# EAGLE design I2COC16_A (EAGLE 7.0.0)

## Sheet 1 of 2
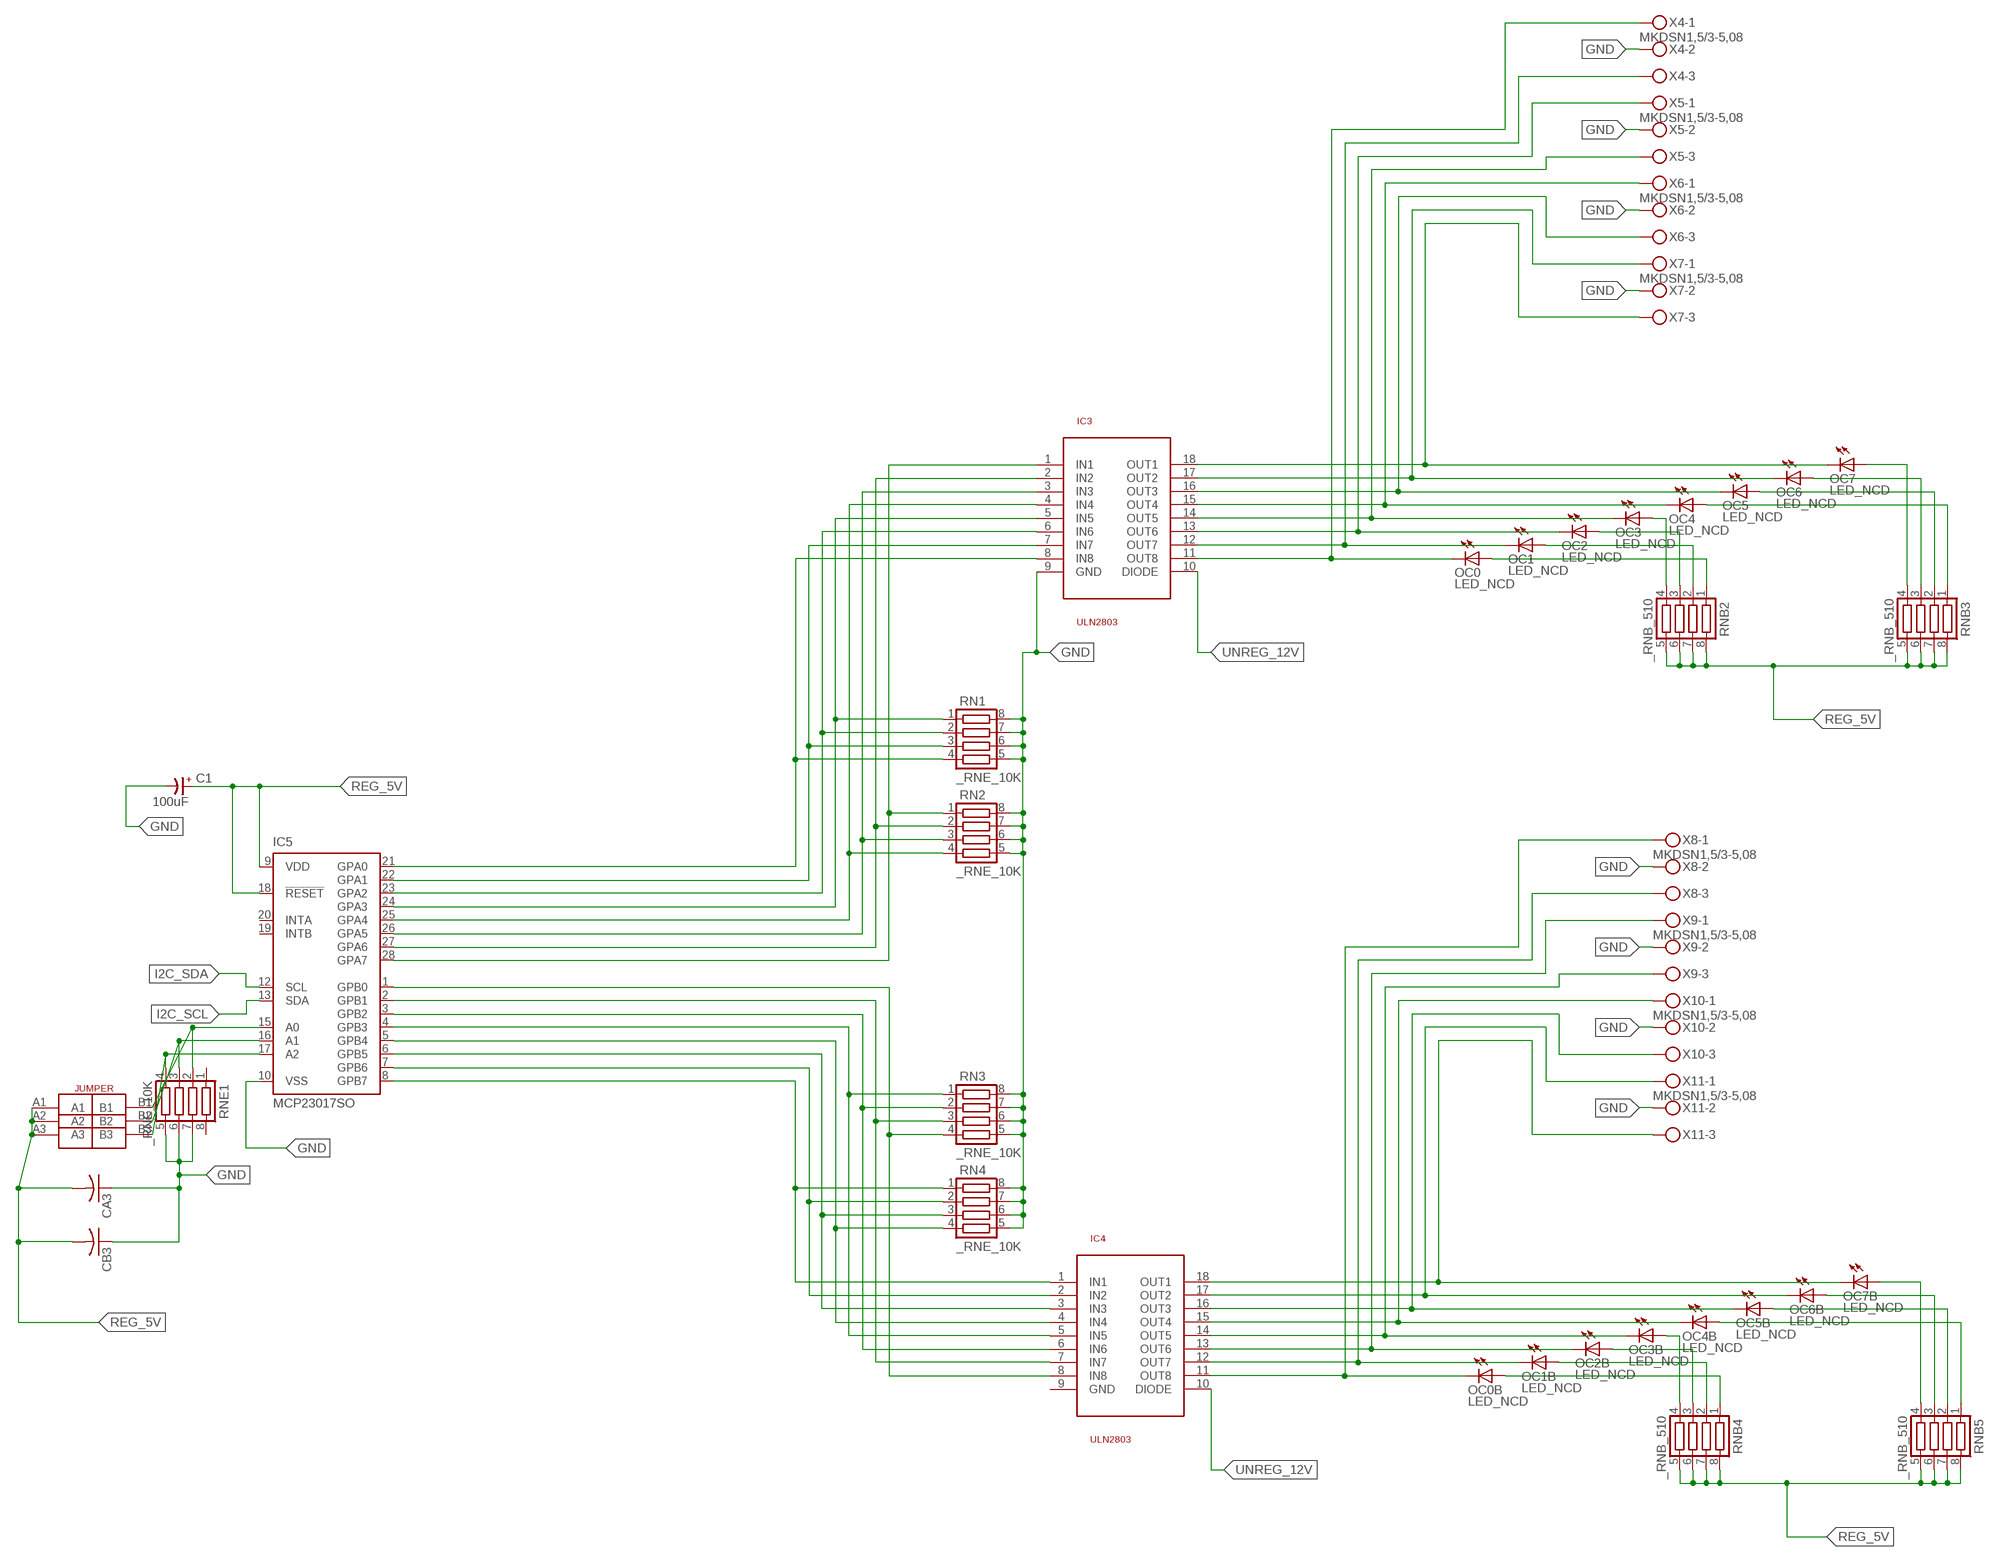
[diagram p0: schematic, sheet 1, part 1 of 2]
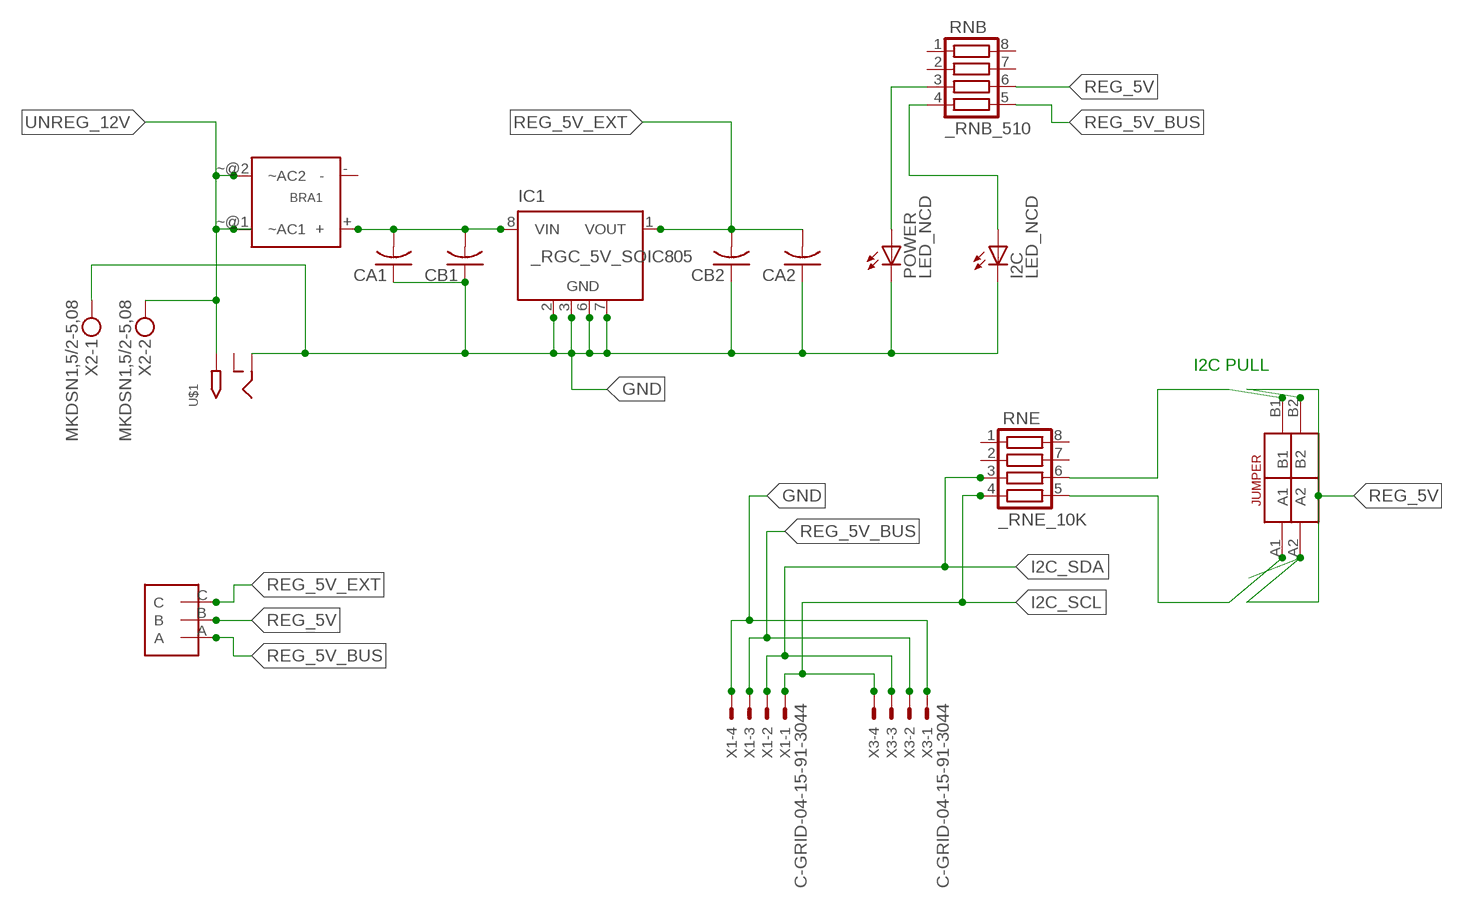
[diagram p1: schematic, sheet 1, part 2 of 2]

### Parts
BRA1  MB2S_  [MB2S]
C1  100uF  CP-E-025X060  [E-025X060]
CA1  CC1206KRX7R9BB104C1206K  [CC1206KRX7R9BB104]
CA2  CC1206KRX7R9BB104C1206K  [CC1206KRX7R9BB104]
CA3  CC1206KRX7R9BB104C1206K  [CC1206KRX7R9BB104]
CB1  TMK316F106ZL-TC1206K  [TMK316F106ZL-T]
CB2  TMK316F106ZL-TC1206K  [TMK316F106ZL-T]
CB3  TMK316F106ZL-TC1206K  [TMK316F106ZL-T]
I2C  LED_NCD  [CHIPLED_0603]
IC1  _RGC_5V_SOIC805  [_RGC_5V_SOIC8]
IC3  ULN2803  [SO18L]
IC4  ULN2803  [SO18L]
IC5  MCP23017SO  [SO28W]
OC0  LED_NCD  [CHIPLED_0603]
OC0B  LED_NCD  [CHIPLED_0603]
OC1  LED_NCD  [CHIPLED_0603]
OC1B  LED_NCD  [CHIPLED_0603]
OC2  LED_NCD  [CHIPLED_0603]
OC2B  LED_NCD  [CHIPLED_0603]
OC3  LED_NCD  [CHIPLED_0603]
OC3B  LED_NCD  [CHIPLED_0603]
OC4  LED_NCD  [CHIPLED_0603]
OC4B  LED_NCD  [CHIPLED_0603]
OC5  LED_NCD  [CHIPLED_0603]
OC5B  LED_NCD  [CHIPLED_0603]
OC6  LED_NCD  [CHIPLED_0603]
OC6B  LED_NCD  [CHIPLED_0603]
OC7  LED_NCD  [CHIPLED_0603]
OC7B  LED_NCD  [CHIPLED_0603]
POWER  LED_NCD  [CHIPLED_0603]
RN1  _RNE_10K  [RNE]
RN2  _RNE_10K  [RNE]
RN3  _RNE_10K  [RNE]
RN4  _RNE_10K  [RNE]
RNB  _RNB_510  [RNB]
RNB2  _RNB_510  [RNB]
RNB3  _RNB_510  [RNB]
RNB4  _RNB_510  [RNB]
RNB5  _RNB_510  [RNB]
RNE  _RNE_10K  [RNE]
RNE1  _RNE_10K  [RNE]
U$1  2.1MMJACK  [PJ-102A]
U$2  JUMPER_1X3  [JUMPER_1X3]
U$3  JUMPER_2X2  [JUMPER_2X2]
U$18  JUMPER_3X2  [JUMPER_3X2]
X1  C-GRID-04-15-91-3044  [15-91-04]
X2  MKDSN1,5/2-5,08  [MKDSN1,5/2-5,08]
X3  C-GRID-04-15-91-3044  [15-91-04]
X4  MKDSN1,5/3-5,08  [MKDSN1,5/3-5,08]
X5  MKDSN1,5/3-5,08  [MKDSN1,5/3-5,08]
X6  MKDSN1,5/3-5,08  [MKDSN1,5/3-5,08]
X7  MKDSN1,5/3-5,08  [MKDSN1,5/3-5,08]
X8  MKDSN1,5/3-5,08  [MKDSN1,5/3-5,08]
X9  MKDSN1,5/3-5,08  [MKDSN1,5/3-5,08]
X10  MKDSN1,5/3-5,08  [MKDSN1,5/3-5,08]
X11  MKDSN1,5/3-5,08  [MKDSN1,5/3-5,08]

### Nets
GND: C1.- CA1.1 CA2.1 CA3.1 CB1.1 CB2.1 CB3.1 I2C.C IC1.2(GND) IC1.3(GND) IC1.6(GND) IC1.7(GND) IC3.9(GND) IC5.10(VSS) POWER.C RN1.5 RN1.6 RN1.7 RN1.8 RN2.5 RN2.6 RN2.7 RN2.8 RN3.5 RN3.6 RN3.7 RN3.8 RN4.5 RN4.6 RN4.7 RN4.8 RNE1.5 RNE1.6 RNE1.7 U$1.RING X1.4 X2.1 X3.1 X4.2 X5.2 X6.2 X7.2 X8.2 X9.2 X10.2 X11.2
I2C_SCL: IC5.13(SDA) RNE.4 X1.1 X3.4
I2C_SDA: IC5.12(SCL) RNE.3 X1.2 X3.3
N$1: BRA1.+ CA1.2 CB1.2 IC1.8(VIN)
N$2: POWER.A RNB.3
N$3: I2C.A RNB.4
N$4: RNE.5 U$3.A1
N$5: RNE.6 U$3.B1
N$6: IC5.15(A0) RNE1.2 U$18.B1
N$7: IC5.16(A1) RNE1.3 U$18.B2
N$8: IC5.17(A2) RNE1.4 U$18.B3
N$9: IC3.11(OUT8) OC0.C X4.1
N$10: IC3.12(OUT7) OC1.C X4.3
N$11: IC3.13(OUT6) OC2.C X5.1
N$12: IC3.14(OUT5) OC3.C X5.3
N$13: IC3.1(IN1) IC5.28(GPA7) RN2.1
N$14: IC3.16(OUT3) OC5.C X6.3
N$15: IC3.17(OUT2) OC6.C X7.1
N$16: IC3.18(OUT1) OC7.C X7.3
N$17: IC3.2(IN2) IC5.27(GPA6) RN2.2
N$18: IC3.3(IN3) IC5.26(GPA5) RN2.3
N$19: IC3.4(IN4) IC5.25(GPA4) RN2.4
N$20: IC3.5(IN5) IC5.24(GPA3) RN1.1
N$21: IC3.6(IN6) IC5.23(GPA2) RN1.2
N$22: IC3.7(IN7) IC5.22(GPA1) RN1.3
N$23: IC3.8(IN8) IC5.21(GPA0) RN1.4
N$24: IC3.15(OUT4) OC4.C X6.1
N$25: OC7.A RNB3.4
N$26: OC6.A RNB3.3
N$27: OC5.A RNB3.2
N$28: OC4.A RNB3.1
N$29: OC3.A RNB2.4
N$30: OC2.A RNB2.3
N$31: OC1.A RNB2.2
N$32: OC0.A RNB2.1
N$33: IC4.11(OUT8) OC0B.C X8.1
N$34: IC4.12(OUT7) OC1B.C X8.3
N$35: IC4.13(OUT6) OC2B.C X9.1
N$36: IC4.14(OUT5) OC3B.C X9.3
N$37: IC4.16(OUT3) OC5B.C X10.3
N$38: IC4.17(OUT2) OC6B.C X11.1
N$39: IC4.18(OUT1) OC7B.C X11.3
N$40: IC4.15(OUT4) OC4B.C X10.1
N$41: OC7B.A RNB5.4
N$42: OC6B.A RNB5.3
N$43: OC5B.A RNB5.2
N$44: OC4B.A RNB5.1
N$45: OC3B.A RNB4.4
N$46: OC2B.A RNB4.3
N$47: OC1B.A RNB4.2
N$48: OC0B.A RNB4.1
N$49: IC4.1(IN1) IC5.8(GPB7) RN4.1
N$50: IC4.2(IN2) IC5.7(GPB6) RN4.2
N$51: IC4.3(IN3) IC5.6(GPB5) RN4.3
N$52: IC4.4(IN4) IC5.5(GPB4) RN4.4
N$53: IC4.5(IN5) IC5.4(GPB3) RN3.1
N$54: IC4.6(IN6) IC5.3(GPB2) RN3.2
N$55: IC4.7(IN7) IC5.2(GPB1) RN3.3
N$56: IC4.8(IN8) IC5.1(GPB0) RN3.4
REG_5V: C1.+ CA3.2 CB3.2 IC5.9(VDD) IC5.18(!RESET) RNB2.5 RNB2.6 RNB2.7 RNB2.8 RNB3.5 RNB3.6 RNB3.7 RNB3.8 RNB4.5 RNB4.6 RNB4.7 RNB4.8 RNB5.5 RNB5.6 RNB5.7 RNB5.8 RNB.6 U$2.B U$3.A2 U$3.B2 U$18.A1 U$18.A2 U$18.A3
REG_5V_BUS: RNB.5 U$2.A X1.3 X3.2
REG_5V_EXT: CA2.2 CB2.2 IC1.1(VOUT) U$2.C
UNREG_12V: BRA1.~@1(~AC1) BRA1.~@2(~AC2) IC3.10(DIODE) IC4.10(DIODE) U$1.TIP X2.2
Unconnected: BRA1.- IC1.4(NC) IC1.5(NC) IC4.9(GND) IC5.19(INTB) IC5.20(INTA) RNB.1 RNB.2 RNB.7 RNB.8 RNE1.1 RNE1.8 RNE.1 RNE.2 RNE.7 RNE.8 U$1.RING_SW

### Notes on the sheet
- I2C PULL

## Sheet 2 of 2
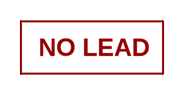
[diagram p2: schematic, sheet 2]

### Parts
U$16  NOPB_LOGO_SYM  [NOPB_LOGO_SYM]

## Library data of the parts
BRA1 = NCD_ULTIMATE_LIBRARY:MB2S: Bridge Rectifier BRA MB2S 200V 500ma Digikey MB2S-TPMSTR-ND/MB2S-TP
C1 = NCD_ULTIMATE_LIBRARY:CP-: Capacitors All Kinds POLARIZED CAP
CA1-CA3 = NCD_ULTIMATE_LIBRARY:CC1206KRX7R9BB104: Capacitor CA .1uF 50V SMT C1206K CC1206KRX7R9BB104
CB1-CB3 = NCD_ULTIMATE_LIBRARY:TMK316F106ZL-T: Capacitor CB 10uF SMT 1206 TMK316F106ZL-T
I2C POWER = NCD_ULTIMATE_bhaskar:LED_NCD
IC1 = NCD_ULTIMATE_LIBRARY:_RGC_5V_SOIC8: Regulator Linear 5V Chip Positive VOLTAGE REGULATOR Digikey 497-7267-2-ND/L78L05CD13TR
IC3 IC4 = NCD_ULTIMATE_LIBRARY:ULN2803: Semiconductor 8 O.C. N-Channel Transistor Driver Digikey ULN2803AFWGCELTR-ND/ULN2803AFWG,C,EL
IC5 = NCD_ULTIMATE_LIBRARY:MCP23017: Semiconductor Port Expander I/O 16-Bit I2C http://ww1.microchip.com/downloads/en/DeviceDoc/21952a.pdf Source: http://ww1.microchip.com/downloads/en/DeviceDoc/21952a.pdf
OC0 OC0B OC1 OC1B OC2 OC2B OC3 OC3B OC4 OC4B OC5 OC5B OC6 OC6B OC7 OC7B = NCD_ULTIMATE_LIBRARY:LED_NCD: LED Digikey 754-1132-2-ND/APT2012SRCPRV
RN1-RN4 RNE RNE1 = NCD_ULTIMATE_LIBRARY:_RNE_10K: Resistor Array RNE SMT 10K x 4 Single Resistor Source: http://www.ctscorp.com/components/Datasheets/CTSChipArrayDs.pdf Digikey 742C083103JPTR-ND/742C083103JP; OC_FARNELL: unknown; OC_NEWARK: unknown
RNB RNB2-RNB5 = NCD_ULTIMATE_LIBRARY:_RNB_510: Resistor Array RNB SMT 510 x 4 Single Resistor Source: http://www.ctscorp.com/components/Datasheets/CTSChipArrayDs.pdf Digikey 742C083511JPTR-ND/ 742C083511JP; OC_FARNELL: unknown; OC_NEWARK: unknown
U$1 = NCD_ULTIMATE_CONNECTORS:2.1MMJACK: 2.1mm x 5.5mm DC jack with internal switch. Digikey part #PJ-102A, 4UCON part #05537 By microbuilder.eu
U$2 = NCD_ULTIMATE_CONNECTORS:JUMPER_1X3
U$3 = NCD_ULTIMATE_CONNECTORS:JUMPER_2X2
U$16 = PatternAgents-Logos:NOPB_LOGO_SYM: NOPB_LOGO_SYM
U$18 = NCD_ULTIMATE_CONNECTORS:JUMPER_3X2
X1 X3 = NCD_ULTIMATE_CONNECTORS:C-GRID-04: CONNECTOR 4-Pos I2C wire to board 2.54 mm (0.100") pitch header Digikey WM1342-ND/0015912045; OC_FARNELL: unknown; OC_NEWARK: unknown
X2 = NCD_ULTIMATE_CONNECTORS:MKDSN1,5/2-5,08: MKDSN 1,5/ 2-5,08 Printklemme
X4-X11 = NCD_ULTIMATE_CONNECTORS:MKDSN1,5/3-5,08: MKDSN 1,5/ 3-5,08 Printklemme Nennstrom: 13,5 A Nennspannung: 250 V Rastermaß: 5,08 mm Polzahl: 3 Anschlussart: Schraubanschluss Montage: Löten Anschlussrichtung Leiter/Platine: 0 ° Artikelnummer: 1729131 Source: http://eshop.phoenixcontact.com .. 1729131.pdf

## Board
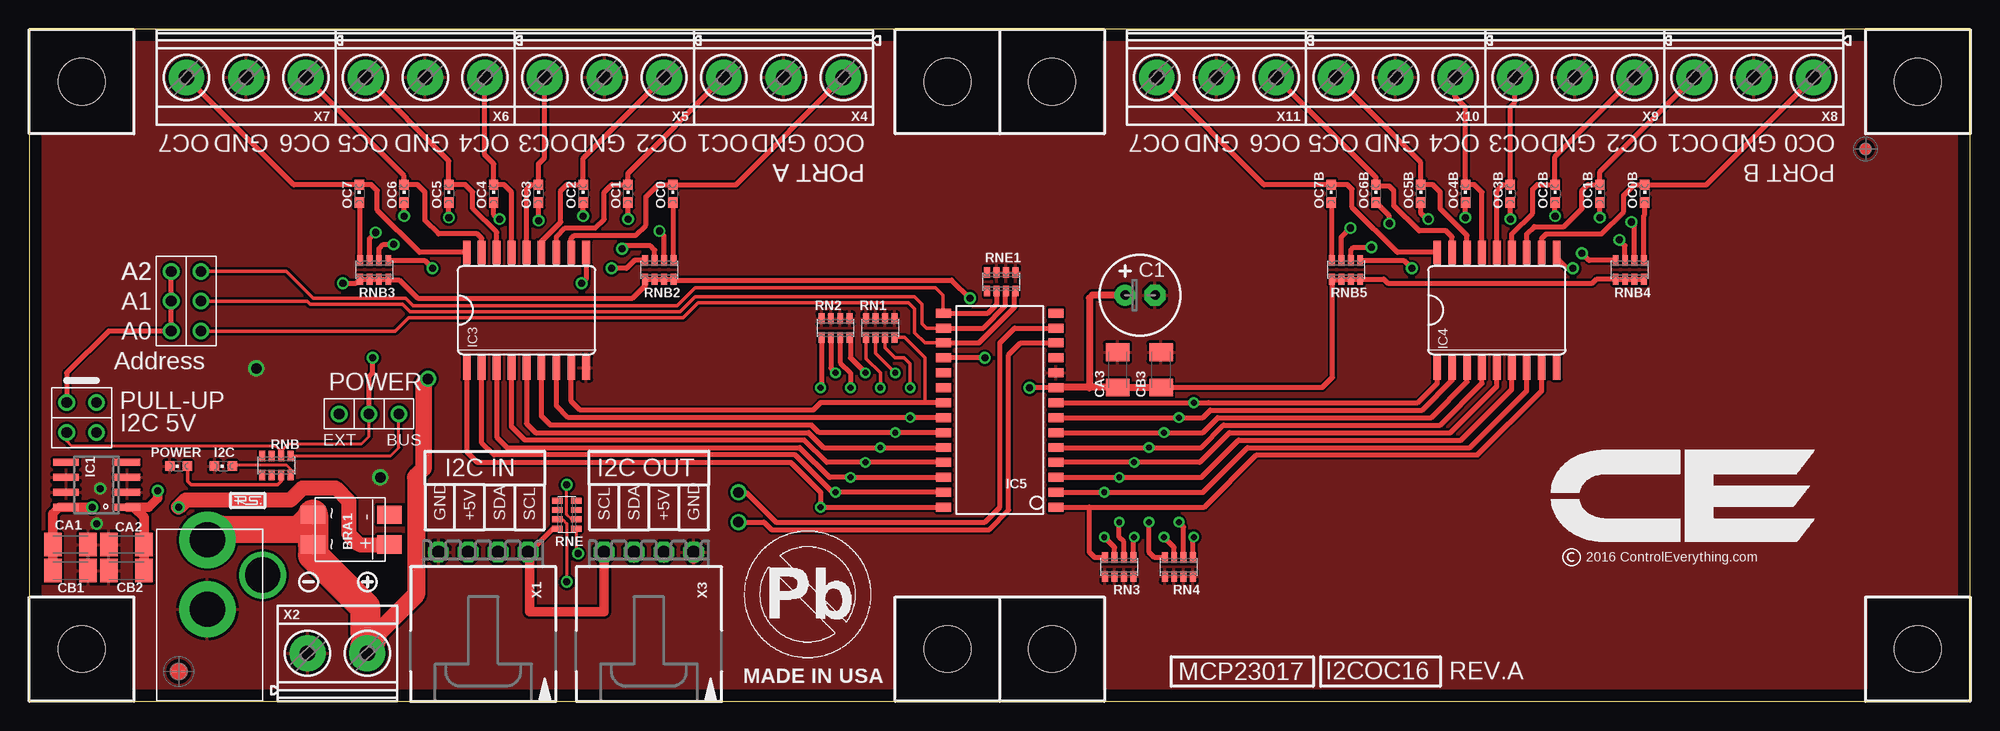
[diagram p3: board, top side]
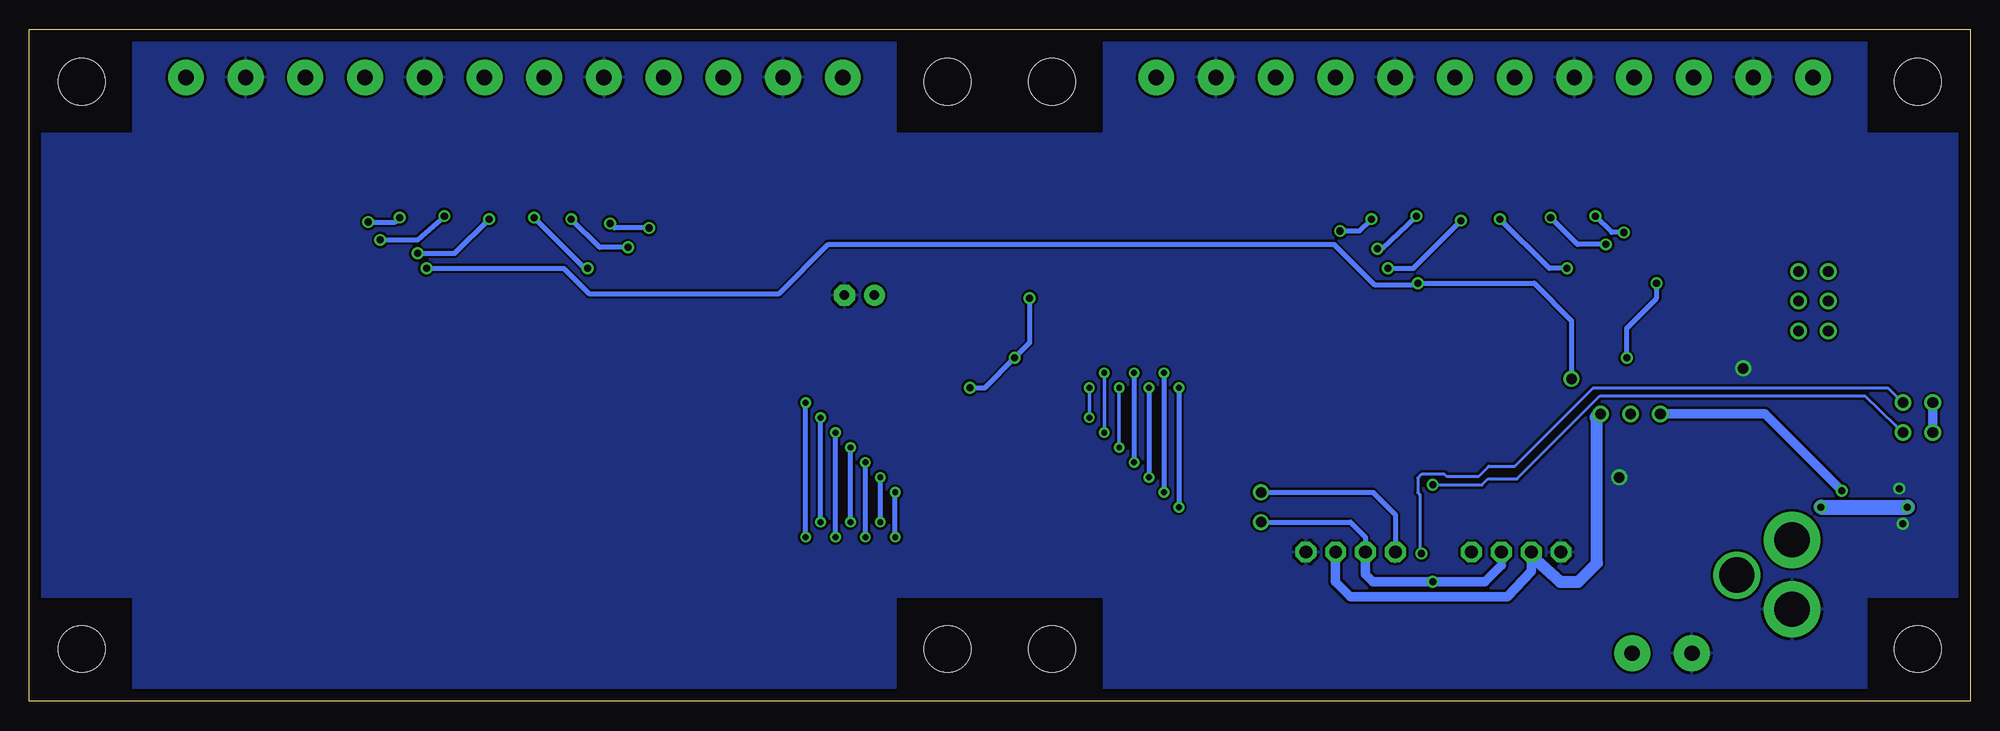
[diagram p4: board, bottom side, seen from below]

Size 165.1 x 57.15 mm. Coordinates in mm from the lower left corner, seen from the top.
Outline: 81.28,0 0,0 0,55.88
Outline: 81.28,0 82.53,0
Outline: 0,56.82 0,55.88
Outline: 81.28,0 82.55,0 163.83,0
Outline: 0,55.88 0,57.15 165.1,57.15 165.1,0 163.83,0
Outline: 163.83,0 165.08,0
Copper layers (1*16): Top 0.035mm / dielectric 1.5mm / Bottom 0.035mm
Design rules "default": minimum track width 10mil, minimum drill 24mil, track to track 8mil, track to pad 8mil, pad to pad 8mil, via to via 8mil, smd to smd 8mil, copper to edge 40mil, drill to drill 8mil, minimum pad ring 10mil, minimum via ring 8mil, stop-mask expansion 4mil, vias tented up to drill 0mil, thermal gap 10mil
Holes 3.96 mm at 4.45,4.45 78.11,4.45 78.11,52.7 4.45,52.7 87,52.7 87,4.45 160.66,4.45 160.66,52.7

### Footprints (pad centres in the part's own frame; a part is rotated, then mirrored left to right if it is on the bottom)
MB2S = smd 1.55 x 2.1: + 0,-6.5; - 2.54,-6.5; ~@1 0,0; ~@2 2.54,0
E-025X060 = drill 0.813 pad 1.778: + -1.27,0 | drill 0.813 pad 1.778 octagon: - 1.27,0
CC1206KRX7R9BB104 = smd 1.5 x 2: 1 -1.5,0; 2 1.5,0
TMK316F106ZL-T = smd 1.5 x 2: 1 -1.5,0; 2 1.5,0
CHIPLED_0603 = smd 0.8 x 0.8: A 0,-0.75; C 0,0.75
_RGC_5V_SOIC8 = smd 0.6 x 2.2: 1 -1.905,-2.6; 2 -0.635,-2.6; 3 0.635,-2.6; 4 1.905,-2.6; 5 1.905,2.6; 6 0.635,2.6; 7 -0.635,2.6; 8 -1.905,2.6
SO18L = smd 0.66 x 2.032: 1 -5.08,-4.902; 2 -3.81,-4.902; 3 -2.54,-4.902; 4 -1.27,-4.902; 5 0,-4.902; 6 1.27,-4.902; 7 2.54,-4.902; 8 3.81,-4.902; 9 5.08,-4.902; 10 5.08,4.902; 11 3.81,4.902; 12 2.54,4.902; 13 1.27,4.902; 14 0,4.902; 15 -1.27,4.902; 16 -2.54,4.902; 17 -3.81,4.902; 18 -5.08,4.902
SO28W = smd 0.762 x 1.27: 1 -7.62,-4.78; 2 -6.35,-4.78; 3 -5.08,-4.78; 4 -3.81,-4.78; 5 -2.54,-4.78; 6 -1.27,-4.78; 7 0,-4.78; 8 1.27,-4.78; 9 2.54,-4.78; 10 3.81,-4.78; 11 5.08,-4.78; 12 6.35,-4.78; 13 7.62,-4.78; 14 8.89,-4.78; 15 8.89,4.78; 16 7.62,4.78; 17 6.35,4.78; 18 5.08,4.78; 19 3.81,4.78; 20 2.54,4.78; 21 1.27,4.78; 22 0,4.78; 23 -1.27,4.78; 24 -2.54,4.78; 25 -3.81,4.78; 26 -5.08,4.78; 27 -6.35,4.78; 28 -7.62,4.78
CHIPLED_0603' = smd 0.8 x 0.876: A 0,-0.75; C 0,0.75
RNE = smd 0.5 x 0.9: 1 -1.2,-0.8; 2 -0.4,-0.8; 3 0.4,-0.8; 4 1.2,-0.8; 5 1.2,0.8; 6 0.4,0.8; 7 -0.4,0.8; 8 -1.2,0.8
RNB = smd 0.5 x 0.9: 1 -1.2,-0.8; 2 -0.4,-0.8; 3 0.4,-0.8; 4 1.2,-0.8; 5 1.2,0.8; 6 0.4,0.8; 7 -0.4,0.8; 8 -1.2,0.8
PJ-102A = drill 3 pad 4.8: RING 0.1,-3.39; TIP 0.1,-9.29 | drill 3 pad 3.251: RING_SW -4.6,-6.29
JUMPER_1X3 = drill 0.9: A 0,5.08; B 0,2.54; C 0,0
JUMPER_2X2 = drill 0.9: A1 0,2.54; A2 0,0; B1 2.54,2.54; B2 2.54,0
JUMPER_3X2 = drill 0.9: A1 0,5.08; A2 0,2.54; A3 0,0; B1 2.54,5.08; B2 2.54,2.54; B3 2.54,0
15-91-04 = drill 1.1 pad 1.778 octagon: 1 -3.81,-7.62; 2 -1.27,-7.62; 3 1.27,-7.62; 4 3.81,-7.62
MKDSN1,5/2-5,08 = drill 1.3 pad 3.048: 1 -2.561,0.025; 2 2.519,0.025
MKDSN1,5/3-5,08 = drill 1.3 pad 3.048: 1 -7.641,0.025; 2 -2.561,0.025; 3 2.519,0.025

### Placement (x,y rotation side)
BRA1  24.13,13.34 90 top
C1  94.49,34.54 0 top
CA1  3.49,13.34 180 top
CA2  8.26,13.34 0 top
CA3  92.58,28.19 270 top
CB1  3.49,11.11 180 top
CB2  8.26,11.11 0 top
CB3  96.27,28.19 270 top
I2C  16.51,20 90 top
IC1  5.71,18.41 90 top
IC3  42.29,33.27 0 top
IC4  124.84,33.27 0 top
IC5  82.55,24.13 90 top
OC0  LED_NCD  [CHIPLED_0603']  54.74,43.18 0 top
OC0B  LED_NCD  [CHIPLED_0603']  137.41,43.18 0 top
OC1  LED_NCD  [CHIPLED_0603']  50.93,43.18 0 top
OC1B  LED_NCD  [CHIPLED_0603']  133.6,43.18 0 top
OC2  LED_NCD  [CHIPLED_0603']  47.12,43.18 0 top
OC2B  LED_NCD  [CHIPLED_0603']  129.79,43.18 0 top
OC3  LED_NCD  [CHIPLED_0603']  43.31,43.18 0 top
OC3B  LED_NCD  [CHIPLED_0603']  125.98,43.18 0 top
OC4  LED_NCD  [CHIPLED_0603']  39.5,43.18 0 top
OC4B  LED_NCD  [CHIPLED_0603']  122.17,43.18 0 top
OC5  LED_NCD  [CHIPLED_0603']  35.69,43.18 0 top
OC5B  LED_NCD  [CHIPLED_0603']  118.36,43.18 0 top
OC6  LED_NCD  [CHIPLED_0603']  31.88,43.18 0 top
OC6B  LED_NCD  [CHIPLED_0603']  114.55,43.18 0 top
OC7  LED_NCD  [CHIPLED_0603']  28.07,43.18 0 top
OC7B  LED_NCD  [CHIPLED_0603']  110.74,43.18 0 top
POWER  12.7,20 90 top
RN1  72.39,31.75 0 top
RN2  68.58,31.75 0 top
RN3  92.71,11.43 180 top
RN4  97.79,11.43 180 top
RNB  21.02,20.07 0 top
RNB2  53.59,36.7 180 top
RNB3  29.34,36.7 180 top
RNB4  136.14,36.7 180 top
RNB5  112.01,36.7 180 top
RNE  45.72,15.88 270 top
RNE1  82.68,35.69 0 top
U$1  15.24,4.45 180 top
U$2  26.35,24.45 270 top
U$3  3.17,25.4 270 top
U$10  [VISION_REF15]  12.7,2.54 0 top
U$16  60.6,3.25 0 top
U$18  12.06,31.5 0 top
U$19  [VISION_REF10]  156.21,46.99 0 top
U$21  [ICON_USA]  60.71,1.52 0 top
U$22  [ICON_MINUS]  23.75,10.16 180 top
U$24  [ICON_PLUS]  28.77,10.16 90 top
X1  38.61,5.08 180 top
X2  26.23,4.06 0 top
X3  52.7,5.08 180 top
X4  61.59,53.09 180 top
X5  46.35,53.09 180 top
X6  31.11,53.09 180 top
X7  15.88,53.09 180 top
X8  144.15,53.09 180 top
X9  128.91,53.09 180 top
X10  113.67,53.09 180 top
X11  98.42,53.09 180 top

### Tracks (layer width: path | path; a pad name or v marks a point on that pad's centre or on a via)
GND  (via drill 0.6, 0.9)
  Top 0.406: 34.8,12.38 X1.4
  Top 0.813: X3.1 56.52,12.06
  other vias: 5.71,15.11 6.03,18.1 19.3,28.32 29.84,19.05
  pour Bottom: -3.17,8.89 8.89,8.89 8.89,-3.17 73.66,-3.17 73.66,8.89 91.44,8.89 91.44,-3.17 156.21,-3.17 156.21,8.89 168.91,8.89 168.91,48.26 156.21,48.26 156.21,60.96 91.44,60.96 91.44,48.26 73.66,48.26 73.66,60.96 8.89,60.96 8.89,48.26 -4.45,48.26 -4.45,8.89
  pour Top: -1.27,48.26 8.89,48.26 8.89,58.42 73.66,58.42 73.66,48.26 91.44,48.26 91.44,58.42 156.21,58.42 156.21,48.26 166.37,48.26 166.37,8.89 156.21,8.89 156.21,-1.27 91.44,-1.27 91.44,8.89 73.66,8.89 73.66,-1.27 8.89,-1.27 8.89,8.89 -1.27,8.89
I2C_SCL  (via drill 0.9)
  Top 0.406: RNE.4 44.51,14.68 42.55,12.7 | v60.33,17.78 60.96,17.78 63.5,15.24 81.28,15.24 82.55,16.51 82.55,30.48 83.82,31.75 IC5.13
  Top 0.813: X3.4 48.9,7.62 42.55,7.62 42.55,12.7 X1.1
  Bottom 0.406: v60.33,17.78 50.8,17.78 48.9,15.88 X3.4
  Bottom 0.61: 48.9,12.06 X3.4
I2C_SDA  (via drill 0.6, 0.9)
  Top 0.254: RNE.3 45.36,15.47 45.72,15.11 v45.72,10.16
  Top 0.406: v60.33,15.24 62.48,15.24 63.12,14.61 81.66,14.61 83.31,16.26 83.31,29.46 84.33,30.48 IC5.12
  Top 0.61: X3.3 51.44,12.06
  Bottom 0.406: v60.33,15.24 52.7,15.24 51.44,13.97 X3.3 51.44,12.06
  Bottom 0.61: 39.88,11.56 X1.2
  Bottom 0.813: 39.88,11.56 41.27,10.16 v45.72,10.16 50.8,10.16 51.44,10.79 51.44,12.06
N$1  (via drill 0.6)
  Top 0.813: CB1.2 CA1.2 1.99,15.96 2.54,16.51 IC1.8 v5.33,16.51
  Top 1.27: v12.7,16.51 13.34,17.14 22.23,17.14 23.24,18.16 26.04,18.16 27.18,17.02 27.18,14.22 28.07,13.34 BRA1.+
  Bottom 1.27: v12.7,16.51 v5.33,16.51
N$2
  Top 0.305: RNB.3 21.4,18.95 21.4,18.7 21.12,18.41 13.78,18.41 13.45,18.74 POWER.A
N$3
  Top 0.254: 22.23,18.95 22.23,19.74 21.9,20.07 16.94,20.07
  Top 0.305: RNB.4 22.23,18.95 | 16.94,20.07 I2C.A
N$4  (via drill 0.6)
  Top 0.254: RNE.5 46.52,12.6 v46.67,12.57
  Bottom 0.254: U$3.A1 6.99,26.67 32.07,26.67 38.73,20 40.96,20 41.85,19.11 44.51,19.11 44.7,19.3 46.67,19.3 46.99,18.99 46.99,17.78 46.8,17.59 46.8,12.7 v46.67,12.57
N$5  (via drill 0.6)
  Top 0.254: RNE.6 46.12,15.47 45.72,15.88 v45.72,18.41
  Bottom 0.254: v45.72,18.41 41.53,18.41 41.02,18.92 38.54,18.92 31.5,25.97 8.95,25.97 6.35,23.5 U$3.B1
N$6
  Top 0.305: U$18.B1 21.84,36.58 24.13,34.29 32,34.29 32.64,33.66 55.12,33.66 56.64,35.18 77.09,35.18 77.72,34.54 77.72,33.07 IC5.15
  Top 0.406: IC5.15 81.53,33.02 82.3,33.78 82.3,34.87 RNE1.2
N$7
  Top 0.305: U$18.B2 23.62,34.04 23.88,33.78 31.75,33.78 32.38,33.15 55.37,33.15 56.64,34.42 75.31,34.42 75.95,33.78 75.95,32.13 76.33,31.75 IC5.16
  Top 0.406: IC5.16 81.15,31.75 83.06,33.66 83.06,34.87 RNE1.3
N$8
  Top 0.305: U$18.B3 31.11,31.5 32.26,32.64 55.63,32.64 56.9,33.91 74.8,33.91 75.31,33.4 75.31,31.37 76.2,30.48 IC5.17
  Top 0.406: IC5.17 80.77,30.48 83.82,33.53 83.82,34.83 RNE1.4
N$9
  Top 0.406: IC3.11 46.1,39.37 46.35,39.62 51.56,39.62 52.45,40.51 52.45,42.93 53.47,43.94 54.73,43.94 OC0.C 60.1,43.93 X4.1
N$10
  Top 0.406: IC3.12 44.83,39.5 45.59,40.26 48.13,40.26 48.9,41.02 48.9,43.31 49.53,43.94 50.91,43.94 OC1.C 50.93,44.91 X4.3
N$11
  Top 0.406: IC3.13 43.56,39.12 45.21,40.77 45.21,43.43 45.72,43.94 47.1,43.94 OC2.C 47.12,46.18 X5.1
N$12
  Top 0.406: IC3.14 42.29,43.56 42.67,43.94 43.3,43.94 OC3.C 43.31,45.72 43.81,46.23 43.81,53.04 X5.3
N$13  (via drill 0.5)
  Top 0.406: IC3.1 37.21,21.21 38.1,20.32 64.77,20.32 67.31,17.78 v67.31,16.51 IC5.28 | RN2.1 67.38,26.74 v67.31,26.67
  Bottom 0.406: v67.31,26.67 v67.31,16.51
N$14
  Top 0.406: IC3.16 39.75,39.88 37.72,41.91 37.72,43.31 37.08,43.94 35.7,43.94 OC5.C 35.69,45.97 X6.3
N$15
  Top 0.406: IC3.17 38.48,39.37 38.1,39.75 34.8,39.75 33.66,40.89 33.66,43.31 33.02,43.94 31.89,43.94 OC6.C 31.88,44.7 X7.1
N$16
  Top 0.406: IC3.18 33.2,38.18 29.59,41.78 29.59,43.43 29.08,43.94 28.08,43.94 OC7.C 22.49,43.93 X7.3
N$17  (via drill 0.5)
  Top 0.406: IC5.27 v68.58,17.78 68.33,17.78 65.15,20.95 39.5,20.95 38.48,21.97 IC3.2 | RN2.2 68.18,28.34 v68.58,27.94
  Bottom 0.406: v68.58,27.94 v68.58,17.78
N$18  (via drill 0.5)
  Top 0.406: IC3.3 39.75,22.48 40.64,21.59 65.53,21.59 68.07,19.05 v69.85,19.05 IC5.26 | RN2.3 68.98,28.81 69.85,27.94 v69.85,26.67
  Bottom 0.406: v69.85,26.67 v69.85,19.05
N$19  (via drill 0.5)
  Top 0.406: IC5.25 v71.12,20.32 67.82,20.32 65.91,22.23 42.16,22.23 41.02,23.37 IC3.4 | RN2.4 69.85,30.95 69.85,29.21 v71.12,27.94
  Bottom 0.406: v71.12,27.94 v71.12,20.32
N$20  (via drill 0.5)
  Top 0.305: RN1.1 71.19,29.14 72.39,27.94 v72.39,26.67
  Top 0.406: IC3.5 42.29,23.62 43.05,22.86 66.29,22.86 67.56,21.59 v72.39,21.59 IC5.24
  Bottom 0.305: v72.39,26.67 v72.39,21.59
N$21  (via drill 0.5)
  Top 0.305: RN1.2 71.99,29.61 v73.66,27.94
  Top 0.406: IC5.23 v73.66,22.86 67.18,22.86 66.55,23.5 44.32,23.5 43.56,24.26 IC3.6
  Bottom 0.305: v73.66,27.94 v73.66,22.86
N$22  (via drill 0.5)
  Top 0.305: RN1.3 72.79,30.08 73.66,29.21 74.42,29.21 74.93,28.7 v74.93,26.67
  Top 0.406: IC5.22 v74.93,24.13 73.66,24.13 45.85,24.13 44.83,25.15 IC3.7
  Bottom 0.305: v74.93,26.67 v74.93,24.13
N$23
  Top 0.305: RN1.4 74.46,30.95 76.2,29.21 76.2,25.4
  Top 0.406: IC5.21 76.2,25.4 67.31,25.4 66.67,24.77 46.86,24.77 46.1,25.53 IC3.8
N$24
  Top 0.406: IC3.15 41.02,43.31 40.39,43.94 39.51,43.94 OC4.C 39.5,45.72 38.73,46.48 38.73,53.04 X6.1
N$25
  Top 0.406: RNB3.4 28.14,42.36 OC7.A
N$26  (via drill 0.6)
  Top 0.406: RNB3.3 28.94,39.35 v29.46,39.88 | v31.88,41.27 OC6.A
  Bottom 0.406: v29.46,39.88 30.48,39.88 v31.88,41.27
N$27  (via drill 0.6)
  Top 0.406: RNB3.2 29.74,38.5 30.1,38.86 v30.99,38.86 | v35.69,41.15 OC5.A
  Bottom 0.406: v30.99,38.86 33.4,38.86 v35.69,41.15
N$28  (via drill 0.6)
  Top 0.406: RNB3.1 33.62,37.5 v34.29,36.83 | v40.01,41.02 39.88,41.02 39.5,41.4 OC4.A
  Bottom 0.406: v34.29,36.83 35.81,36.83 v40.01,41.02
N$29  (via drill 0.6)
  Top 0.406: RNB2.4 51.47,37.5 50.8,36.83 v49.53,36.83 | v43.31,40.89 OC3.A
  Bottom 0.406: v49.53,36.83 47.37,36.83 v43.31,40.89
N$30  (via drill 0.6)
  Top 0.406: RNB2.3 53.19,38.37 52.83,38.73 50.67,38.73 v50.42,38.48 | v47.12,41.27 OC2.A
  Bottom 0.406: v50.42,38.48 50.04,38.48 v47.12,41.27
N$31  (via drill 0.6)
  Top 0.406: RNB2.2 53.99,39.6 v53.59,40.01 | v50.93,41.02 OC1.A
  Bottom 0.406: v53.59,40.01 51.94,40.01 v50.93,41.02
N$32
  Top 0.406: RNB2.1 54.79,42.37 OC0.A
N$33
  Top 0.406: IC4.11 128.65,39.37 129.03,39.75 133.73,39.75 135.64,41.66 135.64,43.05 136.53,43.94 137.4,43.94 OC0B.C 142.66,43.93 X8.1
N$34
  Top 0.406: IC4.12 127.38,39.75 128.02,40.39 130.56,40.39 132.08,41.91 132.08,43.43 132.59,43.94 133.59,43.94 OC1B.C 133.6,45.04 X8.3
N$35
  Top 0.406: IC4.13 126.11,39.75 127.89,41.53 127.89,43.56 128.27,43.94 129.78,43.94 OC2B.C 129.79,46.31 X9.1
N$36
  Top 0.406: IC4.14 124.84,43.43 125.35,43.94 125.97,43.94 | 125.97,43.94 OC3B.C | 125.97,43.94 125.97,50.53 126.36,50.93 126.36,53.04 X9.3
N$37
  Top 0.406: IC4.16 122.3,39.62 120.02,41.91 120.02,43.31 119.38,43.94 118.38,43.94 OC5B.C 118.36,45.84 X10.3
N$38
  Top 0.406: IC4.17 121.03,39.5 120.52,40.01 118.24,40.01 116.08,42.16 116.08,43.43 115.7,43.81 114.67,43.81 OC6B.C 114.55,44.57 X11.1
N$39
  Top 0.406: IC4.18 116.38,38.18 112.52,42.04 112.52,43.56 112.14,43.94 110.76,43.94 OC7B.C 105.04,43.93 X11.3
N$40
  Top 0.406: IC4.15 123.57,43.31 122.94,43.94 122.19,43.94 OC4B.C 122.17,50.55 121.28,51.44 121.28,53.04 X10.1
N$41
  Top 0.406: RNB5.4 110.81,42.36 OC7B.A
N$42  (via drill 0.6)
  Top 0.406: RNB5.3 111.61,39.48 v112.39,40.26 | v115.7,40.64 115.7,41.29 OC6B.A
  Bottom 0.406: v112.39,40.26 115.32,40.26 v115.7,40.64
N$43  (via drill 0.6)
  Top 0.406: RNB5.2 112.41,38.37 112.65,38.61 v114.17,38.61 | v119,41.02 118.87,41.02 118.36,41.53 OC5B.A
  Bottom 0.406: v114.17,38.61 116.59,38.61 v119,41.02
N$44  (via drill 0.6)
  Top 0.406: RNB5.1 116.93,37.5 v117.6,36.83 | v122.17,41.15 OC4B.A
  Bottom 0.406: v117.6,36.83 117.86,36.83 v122.17,41.15
N$45  (via drill 0.6)
  Top 0.406: RNB4.4 132.68,37.5 v132.08,38.1 | v125.98,41.02 OC3B.A
  Bottom 0.406: v132.08,38.1 128.91,38.1 v125.98,41.02
N$46  (via drill 0.6)
  Top 0.406: RNB4.3 135.74,38.75 v135.25,39.24 | v129.79,41.27 OC2B.A
  Bottom 0.406: v135.25,39.24 132.08,39.24 v129.79,41.27
N$47  (via drill 0.6)
  Top 0.406: RNB4.2 136.54,40.49 v136.27,40.77 | v133.6,41.15 OC1B.A
  Bottom 0.406: v136.27,40.77 133.99,40.77 v133.6,41.15
N$48
  Top 0.406: RNB4.1 137.34,41.33 137.41,41.4 OC0B.A
N$49  (via drill 0.5)
  Top 0.406: IC5.8 v99.06,25.4 100.33,25.4 118.11,25.4 119.76,27.05 IC4.1 | RN4.1 98.99,13.9 v99.06,13.97
  Bottom 0.406: v99.06,13.97 v99.06,25.4
N$50  (via drill 0.5)
  Top 0.406: IC5.7 v97.79,24.13 99.82,24.13 100.46,24.77 118.49,24.77 121.03,27.3 IC4.2 | RN4.2 98.19,14.84 v97.79,15.24
  Bottom 0.406: v97.79,15.24 v97.79,24.13
N$51  (via drill 0.5)
  Top 0.406: IC5.6 v96.52,22.86 99.82,22.86 101.09,24.13 119.25,24.13 122.3,27.18 IC4.3 | RN4.3 97.39,13.1 v96.52,13.97
  Bottom 0.406: v96.52,13.97 v96.52,22.86
N$52  (via drill 0.5)
  Top 0.406: IC5.5 v95.25,21.59 99.69,21.59 101.6,23.5 120.02,23.5 123.57,27.05 IC4.4 | RN4.4 95.72,12.23 95.25,12.7 v95.25,15.24
  Bottom 0.406: v95.25,15.24 v95.25,21.59
N$53  (via drill 0.5)
  Top 0.406: IC4.5 124.84,26.8 120.9,22.86 102.11,22.86 99.57,20.32 v93.98,20.32 IC5.4 | RN3.1 93.91,13.9 v93.98,13.97
  Bottom 0.406: v93.98,13.97 v93.98,20.32
N$54  (via drill 0.5)
  Top 0.406: IC5.3 v92.71,19.05 99.69,19.05 102.87,22.23 121.79,22.23 126.11,26.54 IC4.6 | RN3.2 93.11,13.57 92.71,13.97 v92.71,15.24
  Bottom 0.406: v92.71,15.24 v92.71,19.05
N$55  (via drill 0.5)
  Top 0.406: IC5.2 v91.44,17.78 99.82,17.78 103.63,21.59 122.56,21.59 127.38,26.42 IC4.7 | RN3.3 92.31,13.1 v91.44,13.97
  Bottom 0.406: v91.44,13.97 v91.44,17.78
N$56
  Top 0.406: IC5.1 90.17,16.51 | 90.17,16.51 99.95,16.51 104.39,20.95 123.19,20.95 128.65,26.42 IC4.8 | RN3.4 90.64,12.23 90.17,12.7 90.17,16.51
REG_5V  (via drill 0.6)
  Top 0.254: RNB.6 21.42,21.29 | 21.42,21.29 22.04,21.91 28.26,21.91 28.89,22.54 U$2.B | 21.42,21.29 20.99,21.72 3.62,21.72 3.17,22.16 U$3.B2
  Top 0.406: U$18.A1 U$18.A2 U$18.A3 6.73,31.5 3.17,27.94 U$3.A2 | RNB3.8 RNB3.7 RNB3.6 RNB3.5 27.79,35.56 v26.67,35.56 | CB3.2 110.01,26.69 110.87,27.56 110.87,35.85 | 110.87,35.85 RNB5.5 | 110.87,35.85 111.56,35.85 RNB5.6 RNB5.7 RNB5.8 115.23,35.9 115.57,35.56 132.97,35.56 133.35,35.94 134.91,35.94 RNB4.5 RNB4.6 RNB4.7 RNB4.8 | 92.71,26.67 90.17,26.67 IC5.9 v85.09,26.67 | v81.28,29.21 IC5.18 | 30.48,35.85 RNB3.8 | v80.01,34.29 78.47,35.83 54.86,35.83 RNB2.8 RNB2.7 RNB2.6 RNB2.5 52.45,35.85 52.45,35.43 51.31,34.29 33.02,34.29 31.5,35.81 30.63,35.81 RNB3.8 | U$2.B 28.89,27.62 29.21,27.94 v29.21,29.21
  Top 0.61: CB3.2 CA3.2 87.35,26.69 IC5.9 | C1.+ 90.42,34.54 90.17,34.29 90.17,26.67
  Bottom 0.406: v85.09,26.67 83.82,26.67 v81.28,29.21 80.01,30.48 v80.01,34.29 | v29.21,29.21 29.21,31.75 26.67,34.29 v26.67,35.56
  Bottom 0.813: U$3.B2 U$3.A2
REG_5V_BUS
  Top 0.254: U$2.A 31.43,21.59 30.71,20.87 RNB.5
  Top 0.61: X1.3 37.34,12.38 | X3.2 53.98,12.06
  Bottom 0.406: 37.47,12.06 37.34,12.19 37.34,12.38 X1.3 | 53.98,12.06 X3.2
  Bottom 0.813: 37.34,12.38 37.34,11.05 39.37,8.89 52.7,8.89 53.98,10.16 53.98,12.06
  Bottom 1.016: 37.34,12.38 34.86,10.16 33.34,10.16 31.75,11.75 31.75,24.13
  Bottom 1.27: 31.75,24.13 U$2.A
REG_5V_EXT  (via drill 0.6)
  Top 0.813: CB2.2 CA2.2 9.76,15.64 8.89,16.51 | 8.89,16.51 IC1.1 | v10.92,17.91 10.92,17.27 10.16,16.51 8.89,16.51
  Bottom 0.813: v10.92,17.91 17.46,24.45 U$2.C
UNREG_12V  (via drill 0.6, 0.9)
  Top 0.406: IC3.10 47.37,35.94 v46.99,35.56 | IC4.10 129.92,37.72 130.81,36.83 v131.32,36.83
  Top 1.422: 32.89,19.05 32.89,19.18 33.53,19.81 33.53,27.05 v33.91,27.43
  Top 1.524: 32.89,19.05 32.89,9.08 29.11,5.3 28.57,4.76
  Top 2.286: BRA1.~@2 22.86,14.61 16.01,14.61
  Top 2.54: 16.01,14.61 U$1.TIP | X2.2 28.55,4.45 28.57,4.76 | BRA1.~@2 BRA1.~@1 24.13,12.45 28.57,8 28.57,5.84 29.11,5.3
  Bottom 0.406: v33.91,27.43 33.91,32.38 37.08,35.56 v46.99,35.56 47.12,35.43 50.67,35.43 54.1,38.86 97.16,38.86 101.35,34.67 117.47,34.67 119.63,36.83 v131.32,36.83

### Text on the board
tNames: OC7 | GND | OC6 | OC5 | GND | OC4 | OC3 | GND | OC2 | OC1 | GND | OC0 | OC7 | GND | OC6 | OC5 | GND | OC4 | OC3 | GND | OC2 | OC1 | GND | OC0 | PORT A | PORT A | PORT B | A2 | A2 | A1 | A0 | Address | POWER | PULL-UP | I2C 5V | EXT | BUS | I2C IN | I2C OUT | GND | +5V | SDA | SCL | SCL | SDA | +5V | GND | 2016 ControlEverything.com | MCP23017 | I2COC16 | REV.A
